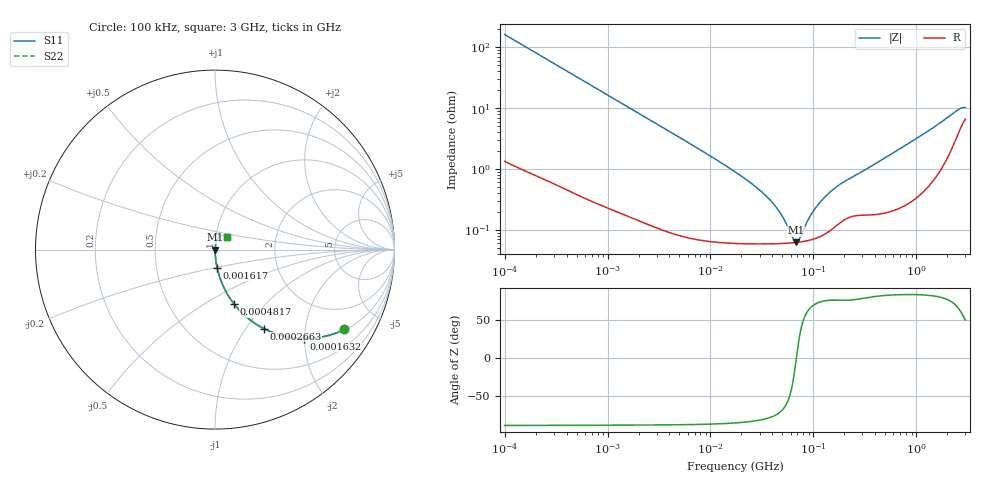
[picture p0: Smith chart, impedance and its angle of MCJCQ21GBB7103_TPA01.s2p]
! MCJCQ21GBB7103_TPA01  S-PARAMETER MODEL  ( Standard Model )
! Model Generated by TAIYO YUDEN Corporation (http://www.ty-top.com)
! Version 1.0
! TAIYO YUDEN Control No. 220601
! Copyright(c) 2015 TAIYO YUDEN CO.,LTD. All Rights Reserved.
! Product Description (link to TY-COMPAS)
! https://ds.yuden.co.jp/TYCOMPAS/or/detail?pn=MCJCQ21GBB7103KTPA01&u=M
! Products Name : Multilayer Ceramic Capacitors
! Characteristics :
!  Capacitance : 0.01 [uF] , Rated Voltage : 250 [V] , TCC : X7R
!  Case Size : 2.0 x 1.25 / 0.079 x 0.049 [mm/inch] , Thickness : 1.25 / 0.049 [mm/inch]
!  (Conditions: Temperature = 25 [degC] , DC Bias Voltage = 0 [V])
! External Node Assignments :
!  1  o---| |---o  2
! GND o---------o GND
! Frequency Range : 100kHz  -  3GHz  [ 401 STEP ]
# MHZ S RI R 50
! Freq[MHz].  S11 Real  S11 Imag  S21 Real  S21 Imag  S12 Real  S12 Imag  S22 Real  S22 Imag
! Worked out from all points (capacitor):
!   401 points, 100 kHz to 3 GHz, reference 50 ohm
!   read as one part in series: C = 9.84 nF near 105.3 kHz
!   lowest |Z| = 62.2 mohm at 67.89 MHz (marker M1)
!   series resonance near 68.41 MHz, so ESL is about 550 pH
!   S11 on the Smith chart (normalised r, x): 100 kHz: 1.03, -3.23; 163.2 kHz: 1.02, -1.98; 266.3 kHz: 1.01, -1.22; 481.7 kHz: 1.01, -0.68; 1.617 MHz: 1.00, -0.20; 3 GHz: 1.13, +0.16
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0.1  0.7213 -0.4442  0.2787 0.4442  0.2787 0.4442  0.7213 -0.4442
0.163179  0.4962 -0.4954  0.5038 0.4954  0.5038 0.4954  0.4962 -0.4954
0.266273  0.2732 -0.4405  0.7268 0.4405  0.7268 0.4405  0.2732 -0.4405
0.481683  0.1055 -0.3015  0.8945 0.3015  0.8945 0.3015  0.1055 -0.3015
0.562235  0.0804 -0.266  0.9196 0.266  0.9196 0.266  0.0804 -0.266
0.941399  0.0315 -0.168  0.9685 0.168  0.9685 0.168  0.0315 -0.168
1.61742  0.0118 -0.1003  0.9882 0.1003  0.9882 0.1003  0.0118 -0.1003
3.161081  0.00375 -0.0519  0.9963 0.0519  0.9963 0.0519  0.00375 -0.0519
17.7727  0.000673 -0.00872  0.9993 0.00872  0.9993 0.00872  0.000673 -0.00872
28.26337  0.000612 -0.00488  0.9994 0.00488  0.9994 0.00488  0.000612 -0.00488
39.51212  0.000598 -0.00281  0.9994 0.00281  0.9994 0.00281  0.000598 -0.00281
48.55934  0.0006 -0.0017  0.9994 0.0017  0.9994 0.0017  0.0006 -0.0017
62.83488  0.000613 -0.000416  0.9994 0.000416  0.9994 0.000416  0.000613 -0.000416
67.88584  0.000621 -3.73e-05  0.9994 3.73e-05  0.9994 3.73e-05  0.000621 -3.73e-05
73.34282  0.00063 0.000342  0.9994 -0.000342  0.9994 -0.000342  0.00063 0.000342
85.60801  0.000659 0.00111  0.9993 -0.00111  0.9993 -0.00111  0.000659 0.00111
97.38194  0.000696 0.00177  0.9993 -0.00177  0.9993 -0.00177  0.000696 0.00177
122.8043  0.000819 0.00305  0.9992 -0.00305  0.9992 -0.00305  0.000819 0.00305
167.3121  0.00119 0.00493  0.9988 -0.00493  0.9988 -0.00493  0.00119 0.00493
547.5153  0.00224 0.0166  0.9978 -0.0166  0.9978 -0.0166  0.00224 0.0166
2441.062  0.0368 0.078  0.9632 -0.078  0.9632 -0.078  0.0368 0.078
3000  0.0664 0.0684  0.9336 -0.0684  0.9336 -0.0684  0.0664 0.0684
